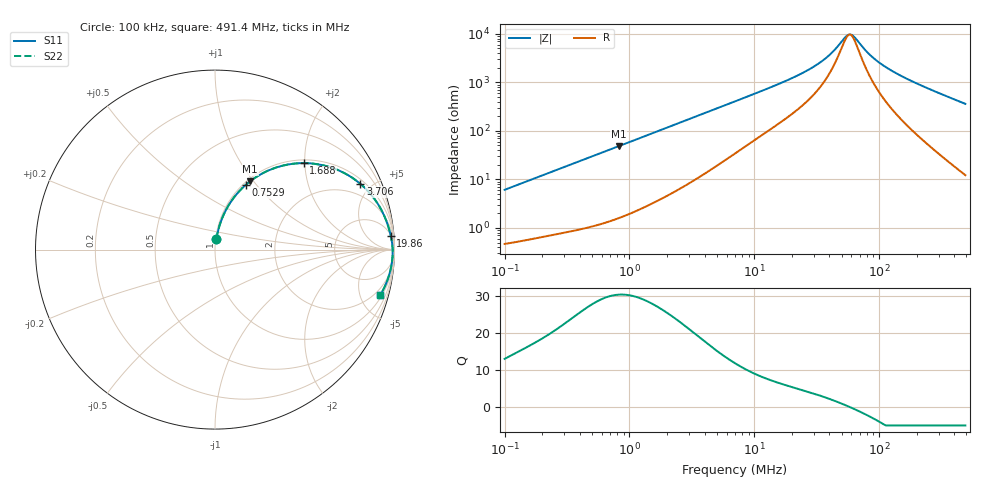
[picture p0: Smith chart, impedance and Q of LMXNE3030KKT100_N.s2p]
! LMXNE3030KKT100_N  S-PARAMETER MODEL  ( General Type )
! Model Generated by TAIYO YUDEN Corporation (https://www.yuden.co.jp/en/)
! Version 1.0
! TAIYO YUDEN Control No. 191023NI43SB-FBB
! Copyright(c) 2019 TAIYO YUDEN CO.,LTD. All Rights Reserved.
! Product Description (link to TY-COMPAS)
! https://ds.yuden.co.jp/TYCOMPAS/or/detail?pn=LMXNE3030KKT100MN&u=M
! Products Name : Inductors
! Characteristics :
!  Inductance : 10 uH , SRF(min) : 34 MHz , DC Resistance(max) : 0.42 Ohm
!  Rated Current : Saturation :600 mA , Temp Rise : 620 mA (40 degC)
!  Case Size : 3.0 x 3.0 / 0.118 x 0.118 [mm/inch] , Thickness : 1 / 0.039 [mm/inch]
!  (Conditions: Temperature = 25 degC , DC Bias Current/Voltage = 0A / 0V)
! External Node Assignments :
!  1  o---GGG---o  2
! GND o---------o GND
! Frequency Range : 0.1MHz  -  491.415554MHz  [ 402 STEP ]
# MHz S RI R 50
! Freq[MHz].  S11 Real  S11 Imag  S21 Real  S21 Imag  S12 Real  S12 Imag  S22 Real  S22 Imag
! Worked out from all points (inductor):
!   401 points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, 100 kHz to 491.4 MHz, reference 50 ohm
!   read as one part in series: L = 9.64 uH near 104.3 kHz
!   highest Q = 30.4 at 819.7 kHz (marker M1), where L = 9.36 uH
!   self-resonance near 57.46 MHz
!   S11 on the Smith chart (normalised r, x): 100 kHz: 1.01, +0.12; 752.9 kHz: 1.03, +0.89; 1.688 MHz: 1.07, +1.97; 3.706 MHz: 1.23, +4.29; 19.86 MHz: 5, +24; 491.4 MHz: 1.24, -7.21
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0.1  0.00828 0.06  0.9917 -0.06  0.9917 -0.06  0.00828 0.06
0.214897  0.0227 0.125  0.9773 -0.125  0.9773 -0.125  0.0227 0.125
0.415258  0.065 0.2279  0.935 -0.2279  0.935 -0.2279  0.065 0.2279
0.752868  0.1724 0.3615  0.8276 -0.3615  0.8276 -0.3615  0.1724 0.3615
0.81966  0.1966 0.3813  0.8034 -0.3813  0.8034 -0.3813  0.1966 0.3813
1.227375  0.346 0.459  0.654 -0.459  0.654 -0.459  0.346 0.459
1.688133  0.4933 0.4818  0.5067 -0.4818  0.5067 -0.4818  0.4933 0.4818
1.72439  0.5035 0.4817  0.4965 -0.4817  0.4965 -0.4817  0.5035 0.4817
2.422665  0.6591 0.4532  0.3409 -0.4532  0.3409 -0.4532  0.6591 0.4532
3.705662  0.8095 0.3668  0.1905 -0.3668  0.1905 -0.3668  0.8095 0.3668
7.010104  0.926 0.2229  0.074 -0.2229  0.074 -0.2229  0.926 0.2229
19.85761  0.979 0.0785  0.021 -0.0785  0.021 -0.0785  0.979 0.0785
29.11  0.9852 0.0467  0.0148 -0.0467  0.0148 -0.0467  0.9852 0.0467
38.37198  0.9879 0.0271  0.0121 -0.0271  0.0121 -0.0271  0.9879 0.0271
44.52609  0.9888 0.0172  0.0112 -0.0172  0.0112 -0.0172  0.9888 0.0172
53.91035  0.9896 0.00481  0.0104 -0.00481  0.0104 -0.00481  0.9896 0.00481
58.69305  0.9898 -0.000662  0.0102 0.000662  0.0102 0.000662  0.9898 -0.000662
63.90004  0.99 -0.00616  0.01 0.00616  0.01 0.00616  0.99 -0.00616
87.88818  0.9897 -0.0276  0.0103 0.0276  0.0103 0.0276  0.9897 -0.0276
120.8815  0.988 -0.0519  0.012 0.0519  0.012 0.0519  0.988 -0.0519
214.552  0.9785 -0.1101  0.0215 0.1101  0.0215 0.1101  0.9785 -0.1101
491.4156  0.9213 -0.2528  0.0787 0.2528  0.0787 0.2528  0.9213 -0.2528
